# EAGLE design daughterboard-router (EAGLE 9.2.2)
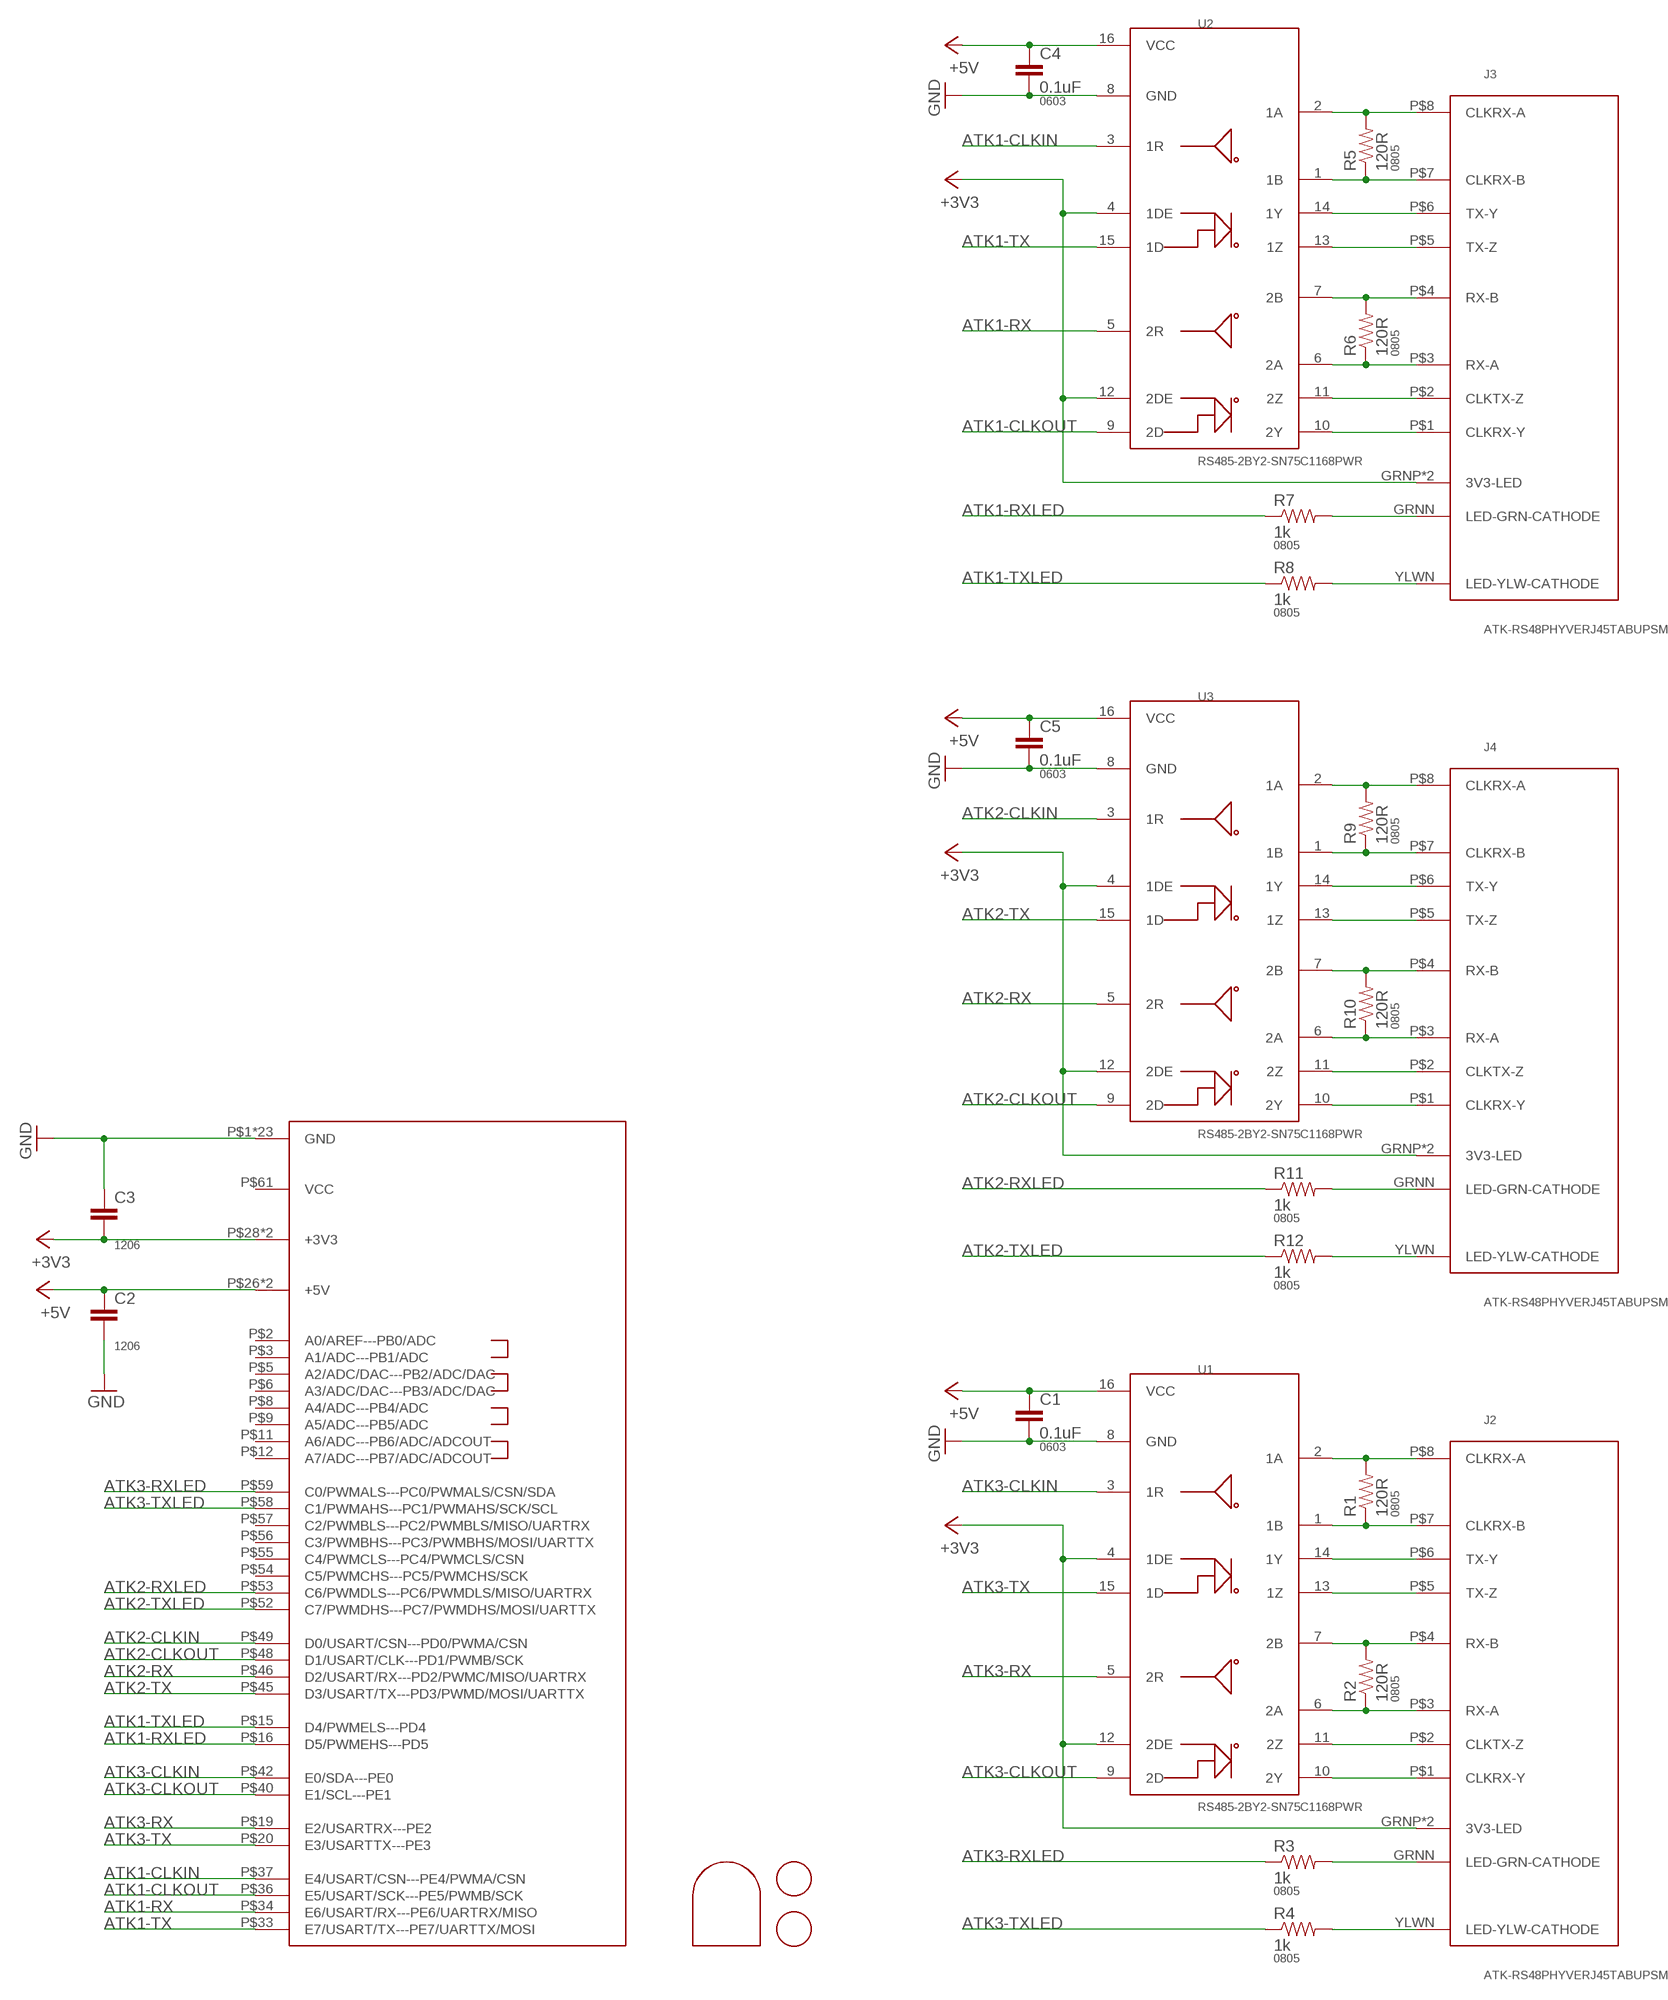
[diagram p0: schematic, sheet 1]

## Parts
C1  0.1uF  CAP0603-CAP  [0603-CAP]
C2  CAP1206  [1206]
C3  CAP1206  [1206]
C4  0.1uF  CAP0603-CAP  [0603-CAP]
C5  0.1uF  CAP0603-CAP  [0603-CAP]
J1  ATK-BFPPFX8-DAUGHTER  [ATK-BFPP-TOP-FX8-60]
J2  ATK-RS48PHYVERJ45TABUPSMD  [RJ45-LED-SMD-RJWURTH-634008137521]
J3  ATK-RS48PHYVERJ45TABUPSMD  [RJ45-LED-SMD-RJWURTH-634008137521]
J4  ATK-RS48PHYVERJ45TABUPSMD  [RJ45-LED-SMD-RJWURTH-634008137521]
J5  FIDUCIALRCT  [FIDUCIAL_RECT_1MM]
J6  FIDUCIALRCT  [FIDUCIAL_RECT_1MM]
MP1  JRTOMBSTONE  [JRTOMBSTONE]
R1  120R  RESISTOR0805-RES  [0805]
R2  120R  RESISTOR0805-RES  [0805]
R3  1k  RESISTOR0805-RES  [0805]
R4  1k  RESISTOR0805-RES  [0805]
R5  120R  RESISTOR0805-RES  [0805]
R6  120R  RESISTOR0805-RES  [0805]
R7  1k  RESISTOR0805-RES  [0805]
R8  1k  RESISTOR0805-RES  [0805]
R9  120R  RESISTOR0805-RES  [0805]
R10  120R  RESISTOR0805-RES  [0805]
R11  1k  RESISTOR0805-RES  [0805]
R12  1k  RESISTOR0805-RES  [0805]
U1  RS485-2BY2-SN75C1168PWR  [TSSOP16]
U2  RS485-2BY2-SN75C1168PWR  [TSSOP16]
U3  RS485-2BY2-SN75C1168PWR  [TSSOP16]

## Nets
+3V3: C3.2 J1.P$28(+3V3) J1.P$29(+3V3) J2.GRNP(3V3-LED) J2.YLWP(3V3-LED) J3.GRNP(3V3-LED) J3.YLWP(3V3-LED) J4.GRNP(3V3-LED) J4.YLWP(3V3-LED) U1.4(1DE) U1.12(2DE) U2.4(1DE) U2.12(2DE) U3.4(1DE) U3.12(2DE)
+5V: C1.1 C2.1 C4.1 C5.1 J1.P$26(+5V) J1.P$27(+5V) U1.16(VCC) U2.16(VCC) U3.16(VCC)
ATK1-CLKIN: J1.P$37(E4/USART/CSN---PE4/PWMA/CSN) U2.3(1R)
ATK1-CLKOUT: J1.P$36(E5/USART/SCK---PE5/PWMB/SCK) U2.9(2D)
ATK1-RX: J1.P$34(E6/USART/RX---PE6/UARTRX/MISO) U2.5(2R)
ATK1-RXLED: J1.P$16(D5/PWMEHS---PD5) R7.1
ATK1-TX: J1.P$33(E7/USART/TX---PE7/UARTTX/MOSI) U2.15(1D)
ATK1-TXLED: J1.P$15(D4/PWMELS---PD4) R8.1
ATK2-CLKIN: J1.P$49(D0/USART/CSN---PD0/PWMA/CSN) U3.3(1R)
ATK2-CLKOUT: J1.P$48(D1/USART/CLK---PD1/PWMB/SCK) U3.9(2D)
ATK2-RX: J1.P$46(D2/USART/RX---PD2/PWMC/MISO/UARTRX) U3.5(2R)
ATK2-RXLED: J1.P$53(C6/PWMDLS---PC6/PWMDLS/MISO/UARTRX) R11.1
ATK2-TX: J1.P$45(D3/USART/TX---PD3/PWMD/MOSI/UARTTX) U3.15(1D)
ATK2-TXLED: J1.P$52(C7/PWMDHS---PC7/PWMDHS/MOSI/UARTTX) R12.1
ATK3-CLKIN: J1.P$42(E0/SDA---PE0) U1.3(1R)
ATK3-CLKOUT: J1.P$40(E1/SCL---PE1) U1.9(2D)
ATK3-RX: J1.P$19(E2/USARTRX---PE2) U1.5(2R)
ATK3-RXLED: J1.P$59(C0/PWMALS---PC0/PWMALS/CSN/SDA) R3.1
ATK3-TX: J1.P$20(E3/USARTTX---PE3) U1.15(1D)
ATK3-TXLED: J1.P$58(C1/PWMAHS---PC1/PWMAHS/SCK/SCL) R4.1
GND: C1.2 C2.2 C3.1 C4.2 C5.2 J1.P$1(GND) J1.P$4(GND) J1.P$7(GND) J1.P$10(GND) J1.P$13(GND) J1.P$14(GND) J1.P$17(GND) J1.P$18(GND) J1.P$21(GND) J1.P$30(GND) J1.P$31(GND) J1.P$32(GND) J1.P$35(GND) J1.P$38(GND) J1.P$39(GND) J1.P$41(GND) J1.P$43(GND) J1.P$44(GND) J1.P$47(GND) J1.P$50(GND) J1.P$51(GND) J1.P$60(GND) J1.P$62(GND) U1.8(GND) U2.8(GND) U3.8(GND)
N$1: J3.P$4(RX-B) R6.2 U2.7(2B)
N$2: J2.P$4(RX-B) R2.2 U1.7(2B)
N$3: J2.P$3(RX-A) R2.1 U1.6(2A)
N$4: J2.P$5(TX-Z) U1.13(1Z)
N$5: J2.P$6(TX-Y) U1.14(1Y)
N$6: J2.P$7(CLKRX-B) R1.1 U1.1(1B)
N$7: J2.P$8(CLKRX-A) R1.2 U1.2(1A)
N$8: J2.P$2(CLKTX-Z) U1.11(2Z)
N$9: J2.P$1(CLKRX-Y) U1.10(2Y)
N$10: J3.P$3(RX-A) R6.1 U2.6(2A)
N$11: J2.GRNN(LED-GRN-CATHODE) R3.2
N$12: J2.YLWN(LED-YLW-CATHODE) R4.2
N$13: J3.P$5(TX-Z) U2.13(1Z)
N$14: J3.P$6(TX-Y) U2.14(1Y)
N$15: J3.P$7(CLKRX-B) R5.1 U2.1(1B)
N$16: J3.P$8(CLKRX-A) R5.2 U2.2(1A)
N$17: J3.P$2(CLKTX-Z) U2.11(2Z)
N$18: J3.P$1(CLKRX-Y) U2.10(2Y)
N$19: J3.GRNN(LED-GRN-CATHODE) R7.2
N$20: J3.YLWN(LED-YLW-CATHODE) R8.2
N$21: J4.P$4(RX-B) R10.2 U3.7(2B)
N$22: J4.P$3(RX-A) R10.1 U3.6(2A)
N$23: J4.P$5(TX-Z) U3.13(1Z)
N$24: J4.P$6(TX-Y) U3.14(1Y)
N$25: J4.P$7(CLKRX-B) R9.1 U3.1(1B)
N$26: J4.P$8(CLKRX-A) R9.2 U3.2(1A)
N$27: J4.P$2(CLKTX-Z) U3.11(2Z)
N$28: J4.P$1(CLKRX-Y) U3.10(2Y)
N$29: J4.GRNN(LED-GRN-CATHODE) R11.2
N$30: J4.YLWN(LED-YLW-CATHODE) R12.2
Unconnected: J1.P$2(A0/AREF---PB0/ADC) J1.P$3(A1/ADC---PB1/ADC) J1.P$5(A2/ADC/DAC---PB2/ADC/DAC) J1.P$6(A3/ADC/DAC---PB3/ADC/DAC) J1.P$8(A4/ADC---PB4/ADC) J1.P$9(A5/ADC---PB5/ADC) J1.P$11(A6/ADC---PB6/ADC/ADCOUT) J1.P$12(A7/ADC---PB7/ADC/ADCOUT) J1.P$54(C5/PWMCHS---PC5/PWMCHS/SCK) J1.P$55(C4/PWMCLS---PC4/PWMCLS/CSN) J1.P$56(C3/PWMBHS---PC3/PWMBHS/MOSI/UARTTX) J1.P$57(C2/PWMBLS---PC2/PWMBLS/MISO/UARTRX) J1.P$61(VCC)

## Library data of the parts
C1 C4 C5 = passives:CAP: Capacitor; PACKAGE: 0603
C2 C3 = passives:CAP: Capacitor; PACKAGE: 1206
J1 = connector:ATK-BFPP
J2-J4 = connector:ATK-RS48PHYVE
J5 J6 = connector:FIDUCIAL: For use by pick and place machines to calibrate the vision/machine, 1mm
MP1 = connector:JRTOMBSTONE
R1-R12 = passives:RESISTOR: Resistor; PACKAGE: 0805
U1-U3 = comm:RS485-2BY2-SN75C1168PWR

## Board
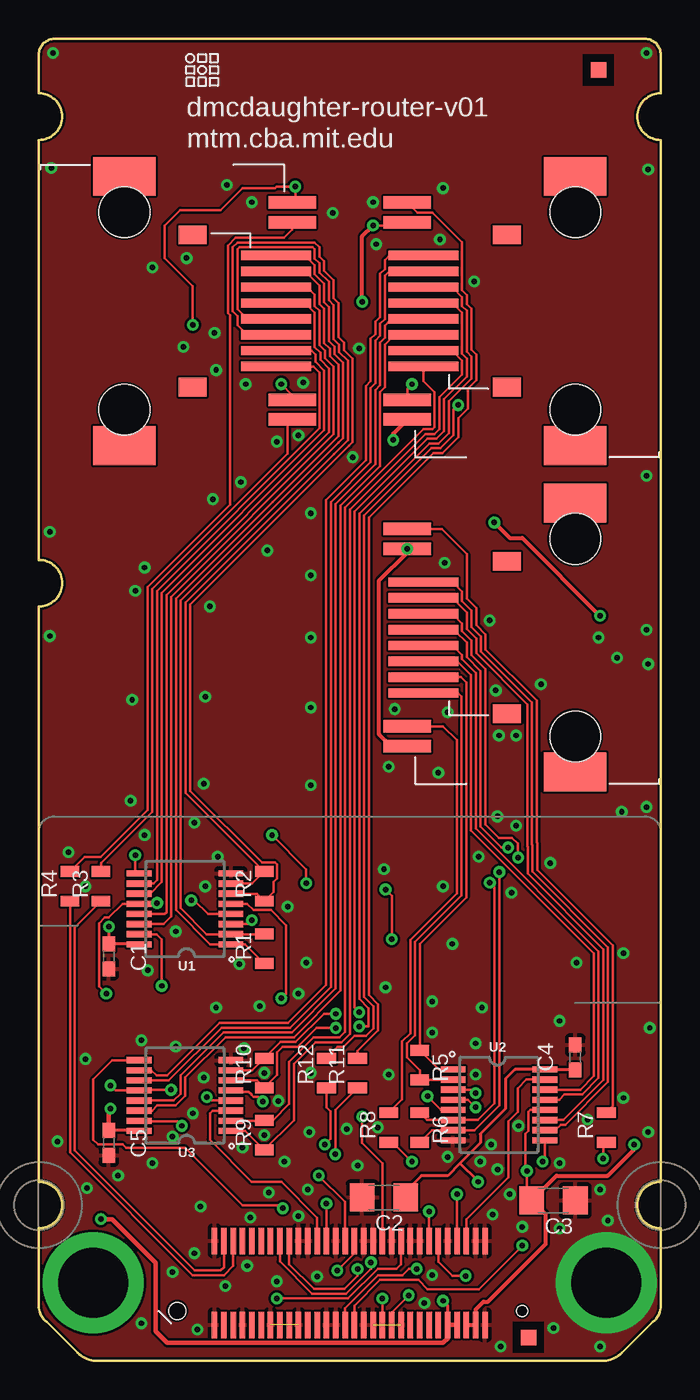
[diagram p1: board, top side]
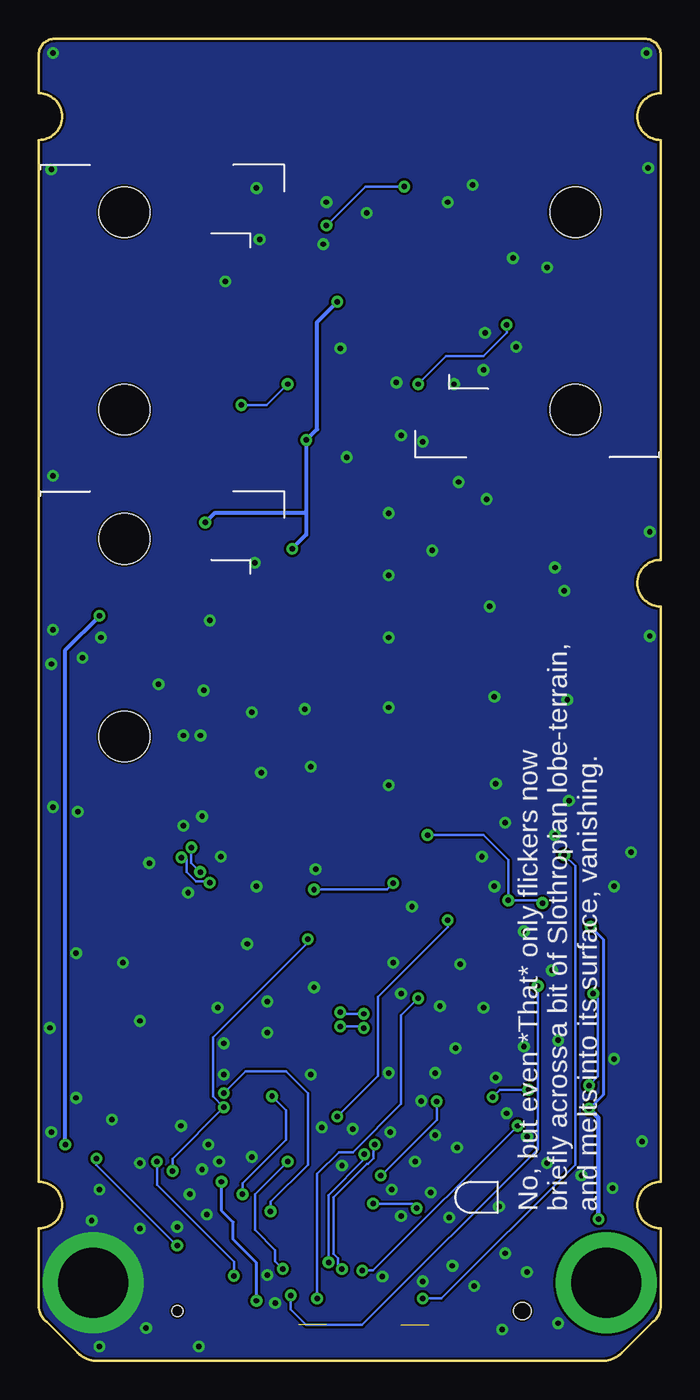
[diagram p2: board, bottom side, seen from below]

Size 40 x 85 mm. Coordinates in mm from the lower left corner, seen from the top.
Outline: 0,3.5 0,8.5 arc90 1.5,10 arc90 0,11.5 0,48.5 arc90 1.5,50 arc90 0,51.5 0,78.5 arc90 1.5,80 arc90 0,81.5 0,84 arc-90 1,85 39,85 arc-90 40,84 40,81.5 arc90 38.5,80 arc90 40,78.5 40,11.5 arc90 38.5,10 arc90 40,8.5 40,3.5 arc-53 39.5,2.5 37.5,0.5 arc-37 36.5,0 3.5,0 arc-37 2.5,0.5 0.5,2.5 arc-53 0,3.5
Copper layers (1*16): Top 0.035mm / dielectric 1.5mm / Bottom 0.035mm
Design rules "default *": minimum track width 6mil, minimum drill 0.35mm, track to track 6mil, track to pad 6mil, pad to pad 6mil, via to via 6mil, smd to smd 6mil, copper to edge 6mil, drill to drill 6mil, minimum pad ring 10mil, minimum via ring 8mil, stop-mask expansion 4mil, vias tented up to drill 30mil, thermal gap 10mil

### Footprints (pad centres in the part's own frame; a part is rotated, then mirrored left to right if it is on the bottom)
0603-CAP = smd 0.96 x 0.8: 1 -0.8,0; 2 0.8,0
1206 = smd 1.6 x 1.8: 1 -1.4,0; 2 1.4,0
ATK-BFPP-TOP-FX8-60 = smd 0.35 x 1.7: P$1 -8.7,-2.7; P$2 -8.1,-2.7; P$3 -7.5,-2.7; P$4 -6.9,-2.7; P$5 -6.3,-2.7; P$6 -5.7,-2.7; P$7 -5.1,-2.7; P$8 -4.5,-2.7; P$9 -3.9,-2.7; P$10 -3.3,-2.7; P$11 -2.7,-2.7; P$12 -2.1,-2.7; P$13 -1.5,-2.7; P$14 -0.9,-2.7; P$15 -0.3,-2.7; P$16 0.3,-2.7; P$17 0.9,-2.7; P$18 1.5,-2.7; P$19 2.1,-2.7; P$20 2.7,-2.7; P$21 3.3,-2.7; P$22 3.9,-2.7; P$23 4.5,-2.7; P$24 5.1,-2.7; P$25 5.7,-2.7; P$26 6.3,-2.7; P$27 6.9,-2.7; P$28 7.5,-2.7; P$29 8.1,-2.7; P$30 8.7,-2.7; P$31 8.7,2.7; P$32 8.1,2.7; P$33 7.5,2.7; P$34 6.9,2.7; P$35 6.3,2.7; P$36 5.7,2.7; P$37 5.1,2.7; P$38 4.5,2.7; P$39 3.9,2.7; P$40 3.3,2.7; P$41 2.7,2.7; P$42 2.1,2.7; P$43 1.5,2.7; P$44 0.9,2.7; P$45 0.3,2.7; P$46 -0.3,2.7; P$47 -0.9,2.7; P$48 -1.5,2.7; P$49 -2.1,2.7; P$50 -2.7,2.7; P$51 -3.3,2.7; P$52 -3.9,2.7; P$53 -4.5,2.7; P$54 -5.1,2.7; P$55 -5.7,2.7; P$56 -6.3,2.7; P$57 -6.9,2.7; P$58 -7.5,2.7; P$59 -8.1,2.7; P$60 -8.7,2.7 | drill 4.5 pad 6.5: P$61 -16.5,0; P$62 16.5,0 | hole 1.1: -11.1,-1.8 | hole 0.7: 11.1,-1.8
RJ45-LED-SMD-RJWURTH-634008137521 = smd 0.8 x 3.05: GRNN 6.98,10.8; GRNP 5.71,10.8; YLWN -5.71,10.8; YLWP -6.98,10.8 | smd 0.6 x 4.5: P$1 3.57,9.76; P$2 2.55,9.76; P$3 1.53,9.76; P$4 0.51,9.76; P$5 -0.51,9.76; P$6 -1.53,9.76; P$7 -2.55,9.76; P$8 -3.57,9.76 | smd 1.2 x 1.8: P$9 -4.9,4.4; P$10 4.9,4.4 | smd 2.5 x 4: P$13 -8.65,0; P$14 8.65,0 | hole 3.25: -6.35,0; 6.35,0
FIDUCIAL_RECT_1MM = smd 1 x 1: P$1 0,0
0805 = smd 0.7 x 1.2: 1 -0.95,0; 2 0.95,0
TSSOP16 = smd 0.4 x 1.6: 1 -2.225,-2.85; 2 -1.575,-2.85; 3 -0.925,-2.85; 4 -0.275,-2.85; 5 0.375,-2.85; 6 1.025,-2.85; 7 1.675,-2.85; 8 2.325,-2.85; 9 2.325,3.05; 10 1.675,3.05; 11 1.025,3.05; 12 0.375,3.05; 13 -0.275,3.05; 14 -0.925,3.05; 15 -1.575,3.05; 16 -2.225,3.05

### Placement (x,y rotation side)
C1  4.5,26 270 top
C2  22.2,10.5 180 top
C3  33.1,10.3 180 top
C4  34.5,19.5 90 top
C5  4.5,14 270 top
J1  20,5 0 top
J2  5.5,67.5 270 top
J3  34.5,46.5 90 top
J4  34.5,67.5 90 top
J5  36,83 0 top
J6  31.5,1.5 0 top
MP1  11.5,10.5 90 bottom
R1  14.5,26.5 90 top
R2  14.5,30.5 90 top
R3  4,30.5 90 top
R4  2,30.5 90 top
R5  24.5,19 270 top
R6  24.5,15 270 top
R7  36.5,15 90 top
R8  22.5,15 90 top
R9  14.5,14.5 90 top
R10  14.5,18.5 90 top
R11  20.5,18.5 90 top
R12  18.5,18.5 90 top
U1  9.5,29 90 top
U2  29.5,16.5 270 top
U3  9.5,17 90 top
U$1  CBA-LOGO  [CBA-SILK-LOGO]  10.5,83 0 top

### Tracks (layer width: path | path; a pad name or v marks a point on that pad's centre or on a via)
+3V3  (via drill 0.35)
  Top 0.152: J2.YLWP 16.5,74.68 v16.5,75.5 15.3,75.5 15.2,75.4 13.1,75.4 11.7,74 9.1,74 8.1,73 8.1,70.9 9.9,69.1 v9.9,66.6 | v21.5,73 23.49,73 J4.GRNP | v7.6,29.43 7.55,29.38 U1.12 5.38,29.38 4.51,28.51 4.25,28.51 3.87,28.13 3.87,24.06 v4.33,23.6 | v9.8,29.6 10,29.6 10.88,28.73 U1.4 | U2.4 27.62,16.77 v28.1,16.29 | C3.2 31.4,10.6 v31.4,12.2 31.3,12.3 31.3,14.57 31.5,14.77 31.5,16 31.62,16.12 U2.12 | U3.4 11.03,16.73 v10.8,16.95 | v4.6,17.7 4.92,17.38 U3.12 6.49,17.42 v8.51,17.42 | v22.7,27.1 22.7,29.9 v22.3,30.3 | v17.2,30.7 17.2,31.6 v15,33.8 | J2.GRNP 16.3,62.1 v15.6,62.8
  Top 0.254: J1.P$28 J1.P$29 28.1,3.3 28.6,3.8 28.9,3.8 32.6,7.5 32.6,9.4 C3.2 33.3,11.9 36.6,11.9 38.3,13.6 v38.3,13.9 | J3.YLWP 22.65,39.52 21.9,40.27 21.9,50.17 23.7,51.98 J3.GRNP | J4.YLWP 22.8,59.62 v22.8,59.2 | v20.8,68.1 20.8,72.3 v21.5,73 | v29.3,53.9 30.3,52.9 31.1,52.9 v36.1,47.9
  Bottom 0.152: v16.5,75.5 19,75.5 v21.5,73 | v7.6,29.43 7.78,29.6 v9.8,29.6 9.8,32.2 11.4,33.8 v15,33.8 | v31.4,12.2 31.4,12.99 v28.1,16.29 28.8,16.99 28.8,20.8 22.7,26.9 v22.7,27.1 | v4.6,17.7 4.03,18.27 4.03,23.3 v4.33,23.6 | v8.51,17.42 10.33,17.42 v10.8,16.95 | v22.3,30.3 17.6,30.3 v17.2,30.7 | v15.6,62.8 13.8,64.6 11.4,64.6 9.9,66.1 v9.9,66.6
  Bottom 0.254: v38.3,13.9 38.3,45.7 v36.1,47.9 | 22.8,54.5 v22.8,59.2 22.1,59.9 22.1,66.8 v20.8,68.1 | 22.8,54.5 22.8,53.11 J3.GRNP | 22.8,54.5 28.7,54.5 v29.3,53.9
  other vias: 23.7,52.21
+5V  (via drill 0.35)
  Top 0.152: 32.58,18.7 U2.16 | 23.6,10.9 C2.1
  Top 0.203: C4.1 32.58,18.7 | U2.16 30.62,18.73 30.03,18.13 30.03,16.2 28.4,14.57 28.4,14 27.1,12.7 | 27.1,12.7 26.3,11.9 24.6,11.9 23.6,10.9 | U3.16 6.42,14.8 C5.1 | v4.5,27.9 C1.1 6.42,26.8 U1.16 | J1.P$26 26.3,3.55 v26,3.85 | v28.25,11.5 28.25,11.55 27.1,12.7
  Top 0.305: J1.P$27 J1.P$26 26.3,1.44 26,1.15 8.26,1.15 7.5,1.9 7.5,6.3 4.7,9.1 v4,9.1 | v4.6,16.2 4.5,16.1 C5.1
  Bottom 0.203: v4.5,27.9 3.7,27.1 3.7,17.1 v4.6,16.2 | v26,3.85 26,6.3 27.5,7.8 27.5,8.9 28.25,9.65 v28.25,11.5
  Bottom 0.305: v4,9.1 4,15.6 v4.6,16.2
ATK1-CLKIN  (via drill 0.35)
  Top 0.152: U2.3 27.88,17.43 v28.1,17.2 | J1.P$37 v25.1,9.6
  Bottom 0.152: v25.1,9.6 25.1,10.2 22.7,12.6 22.7,17.2 24.1,18.6 26.7,18.6 v28.1,17.2
ATK1-CLKOUT  (via drill 0.35)
  Top 0.152: U2.9 32.55,12.95 v32.4,12.8 | J1.P$36 25.7,6.35 26.6,5.45 v27.45,5.45
  Bottom 0.152: v32.4,12.8 32.4,11.3 27.45,6.35 v27.45,5.45
ATK1-RX  (via drill 0.35)
  Top 0.152: U2.5 25.88,16.12 v25,17 | v26.9,10.7 J1.P$34
  Bottom 0.152: v25,17 24.1,16.1 24.1,14.2 26.9,11.4 v26.9,10.7
ATK1-RXLED  (via drill 0.35)
  Top 0.152: J1.P$16 20.3,3.54 21.96,5.2 24.41,5.2 25,4.6 28.3,4.6 v31.1,7.4 | v36.3,13 36.3,13.85 R7.1
  Bottom 0.152: v31.1,7.4 36.3,12.6 v36.3,13
ATK1-TX
  Top 0.152: J1.P$33 27.5,9.1 30.2,11.8 30.2,15.4 30.8,16 30.8,17.5 31.38,18.07 U2.15
ATK1-TXLED  (via drill 0.35)
  Top 0.152: R8.1 22.75,14.05 v24,12.8 | v24.3,5.9 23.8,5.9 23.4,5.5 21.83,5.5 19.7,3.37 J1.P$15
  Bottom 0.152: v24,12.8 26.1,10.7 26.1,8.4 24.8,7.1 24.8,6.4 v24.3,5.9
ATK2-CLKIN
  Top 0.152: U3.3 11.18,16.07 11,15.9 11,14.2 13.7,11.5 15.6,11.5 17.9,9.2 J1.P$49
ATK2-CLKOUT  (via drill 0.35)
  Top 0.152: J1.P$48 v18.5,10.1 | v15.7,9.8 15.5,10 13.1,10 9.4,13.7 5.6,13.7 5.39,13.91 4,13.91 4,13.9 3.8,13.9 3.5,14.2 3.5,18.1 4.72,19.32 U3.9
  Bottom 0.152: v18.5,10.1 16,10.1 v15.7,9.8
ATK2-RX  (via drill 0.35)
  Top 0.152: J1.P$46 19.7,10.2 v18,11.9 | v14.4,16.67 14.1,16.97 13.8,16.97 13.67,17.11 13.67,17.13 13.5,17.3 12.43,17.3 U3.5
  Bottom 0.152: v18,11.9 14.4,15.5 v14.4,16.67
ATK2-RXLED  (via drill 0.35)
  Top 0.152: R11.1 19.07,16.12 v19.07,13.27 | v21.36,6.32 21.36,5.89 19.77,4.3 17.57,4.3 15.5,6.38 J1.P$53
  Bottom 0.152: v19.07,13.27 19.07,12.93 21.36,10.64 v21.36,6.32
ATK2-TX  (via drill 0.35)
  Top 0.152: U3.15 6.47,15.4 8.9,15.4 v9.2,15.1 | v19.2,5.8 20.3,6.9 J1.P$45
  Bottom 0.152: v9.2,15.1 18.5,5.8 v19.2,5.8
ATK2-TXLED  (via drill 0.35)
  Top 0.152: R12.1 18.5,16.3 18.77,16.03 18.77,14.27 v18.4,13.9 | v20.5,5.89 20.5,5.46 19.65,4.61 17.7,4.61 16.1,6.21 J1.P$52
  Bottom 0.152: v18.4,13.9 18.46,13.84 18.46,13.02 18.82,12.66 18.91,12.66 21.06,10.51 21.06,6.87 20.75,6.57 20.75,6.14 v20.5,5.89
ATK3-CLKIN  (via drill 0.35)
  Top 0.152: U1.3 13.44,28.07 v13.7,28.33 | v20.8,15.7 20.8,14 22.1,12.7 J1.P$42
  Bottom 0.152: v13.7,28.33 13.7,27.9 18.2,23.4 18.2,18.3 v20.8,15.7
ATK3-CLKOUT  (via drill 0.35)
  Top 0.152: U1.9 6.2,31.57 v6.2,32.5 | v15.3,4 19.9,4 21.8,5.9 23,5.9 23.3,6.2 J1.P$40
  Bottom 0.152: v6.2,32.5 5.5,31.8 5.5,12.6 14.1,4 v15.3,4
ATK3-RX  (via drill 0.35)
  Top 0.152: J1.P$19 v22.1,4 | v15.6,23.3 15.9,23.6 15.9,28 14.93,28.97 13.8,28.97 13.4,29.38 U1.5
  Bottom 0.152: v15.6,23.3 16.7,22.2 16.7,16.5 19.8,13.4 20.7,13.4 22.1,12 v22.1,4
ATK3-RXLED
  Top 0.152: J1.P$59 11.9,6 11.71,5.8 10.03,5.8 2.31,13.53 2.31,27.86 R3.1
ATK3-TX  (via drill 0.35)
  Top 0.152: U1.15 7.58,27.43 7.9,27.1 v7.9,24.1 | J1.P$20 22.7,3.1 v23.8,4.2
  Bottom 0.152: v7.9,24.1 7.9,13.6 19.2,2.3 22.8,2.3 23.8,3.3 v23.8,4.2
ATK3-TXLED
  Top 0.152: R4.1 2,13.4 9.9,5.5 11.9,5.5 12.5,6.1 J1.P$58
GND  (via drill 0.35)  (2 unrouted)
  other vias: 20.6,65.1 20.2,58.1 26.6,26.8 11.5,32.4 17.5,54.5 17.5,50.5 17.5,46.5 17.5,42 17.5,37 13.2,20.1 15.4,16.7 14.5,18.5 14.5,14.5 17.5,18.5 16.7,23.6 17.2,25.6 19.8,14.9 14.8,10.8 10.4,9.9 7.3,12.7 8.8,20.2 6.6,20.6 30.85,15.1 33.5,21.85 20.5,12.55 10.6,18.2 9.9,15.9 10,6.9 5.1,11.9 3.1,11.1 3,19.4 1.2,14.1 3,30.5 8.8,27.6 10.7,30.5 10,34.6 16,29.2 12.9,25.5 7,25.1 14.2,22.8 22.3,24 22.2,31.6 26,30.5 28.3,32.4 25.3,21.1 28.5,22.7 22.5,18.4 17.4,14.7 13.1,13.7 15.8,12.8 17.3,11 16.7,9.3 13.6,9.2 13.4,6.1 12,4.8 6.6,2.4 10.2,2 17.9,5.4 15.3,5.1 24.8,3.7 25.3,5.5 21.8,15 25.3,23.1 28.1,20.4 28.1,18.4 30.4,30.1 32.9,32 37.6,26.2 37.6,16.9 35.3,15.5 33.5,12.7 36.1,11 39.2,14.7 33.5,8.5 31.1,8.6 33.1,2.1 29.7,0.9 36.1,0.9 36.6,9 29.5,12.3 29.1,13.9 28.4,12.8 26.3,13.1 29.2,9.4 30.3,10.7 8.6,5.7 8.6,14.4 11.4,22.7 5.9,36 1.9,32.7 6.8,33.8 10.6,37.1 6.8,51 6.2,49.5 11,48.5 14.7,52.1 10.7,42.7 6,42.5 11.2,55.4 13.3,62.8 17,62.9 15.3,59.1 13,56.5 28,69.4 25.8,72.1 21.7,71.8 21.5,74.5 26,75.4 18.9,73.8 13.7,74.5 12.1,75.6 9.5,70.9 7.3,70.3 9.3,65.2 11.3,66.1 11.4,63.7 29.4,43.1 29.6,40.2 30.7,34.4 30.7,40.2 29.5,35 26.3,41.7 22.9,41.9 26.1,51.3 16.7,59.5 0.7,46.6 0.7,53.3 0.8,76.7 0.9,84.1 39.1,84.1 39.2,76.6 39.1,56.9 39.1,47 37.2,45.2 39.2,44.8 36,46.5 37.5,35.3 39.1,35.6 39.3,21.4 34.6,25.6 32.3,43.5 29,47.6 25.7,37.8 22.5,38.2
  pour Top: -1,86 41,86 41,-1 -1,-1
  pour Bottom: -2,87 42,87 42,-2 -2,-2
N$1  (via drill 0.35)
  Top 0.152: J3.P$4 24.85,46.9 26.8,46.9 27.52,46.18 27.52,45.24 28.41,44.35 28.41,34.35 29.77,32.99 v30.2,32.99 | v29.62,31.42 29.62,16.42 28.02,14.82 U2.7 25.27,14.82 R6.2
  Bottom 0.152: v30.2,32.99 30.2,32 v29.62,31.42
N$2
  Top 0.152: U1.7 13.72,30.68 R2.2 9.43,36.52 9.43,48.74 18.99,58.3 | J2.P$4 13.4,67 12.78,67.61 12.78,71.47 12.91,71.6 17.61,71.6 17.74,71.47 17.74,70.88 18.04,70.57 18.04,69.98 18.65,69.37 18.65,68.19 18.96,67.89 18.96,65.7 19.32,65.33 19.32,64.86 19.88,64.3 19.88,59.2 18.99,58.3 | 18.99,58.3
N$3
  Top 0.152: U1.6 14.03,30.02 R2.1 15.1,30.15 15.1,30.78 15.33,31 15.33,31.89 15.2,32.03 14.35,32.03 9.73,36.65 9.73,48.62 19.96,58.84 | J2.P$3 13.41,65.97 12.78,66.59 12.78,67.18 12.48,67.49 12.48,71.59 12.79,71.9 17.73,71.9 18.04,71.59 18.04,71 18.35,70.7 18.35,70.11 18.96,69.5 18.96,68.32 19.26,68.02 19.26,65.82 19.63,65.46 19.63,64.99 20.19,64.43 20.19,59.07 19.96,58.84 | 19.96,58.84
N$4
  Top 0.152: U1.13 8.1,28.73 8.21,28.84 8.21,49.25 18.66,59.7 18.66,63.8 18.11,64.36 18.11,64.83 17.74,65.19 17.74,67.39 17.11,68.01 J2.P$5
N$5
  Top 0.152: J2.P$6 17.27,69.03 17.74,68.56 17.74,67.82 18.04,67.51 18.04,65.32 18.41,64.95 18.41,64.48 18.97,63.92 18.97,59.58 8.51,49.12 8.51,28.57 8.02,28.07 U1.14
N$6
  Top 0.152: R1.1 13.28,26.77 U1.1 11.03,26.77 8.82,28.98 8.82,48.99 15.02,55.2 | J2.P$7 17.11,70.05 18.04,69.12 18.04,67.94 18.35,67.64 18.35,65.44 18.71,65.08 18.71,64.61 19.27,64.05 19.27,59.45 15.02,55.2 | 15.02,55.2
N$7
  Top 0.152: R1.2 14.47,27.43 U1.2 10.81,27.43 9.12,29.11 9.12,48.87 19.28,59.02 | J2.P$8 17.11,71.07 17.74,70.44 17.74,69.86 18.35,69.25 18.35,68.07 18.65,67.76 18.65,65.57 19.02,65.2 19.02,64.74 19.58,64.18 19.58,59.32 19.28,59.02 | 19.28,59.02
N$8
  Top 0.152: U1.11 7.16,30.02 7.91,30.77 7.91,49.37 18.36,59.83 18.36,63.67 17.8,64.23 17.8,64.7 17.55,64.95 J2.P$2
N$9
  Top 0.152: J2.P$1 17.67,63.93 18.05,63.55 18.05,59.95 7.6,49.5 7.6,30.9 7.38,30.68 U1.10
N$10  (via drill 0.35)
  Top 0.152: R6.1 24.98,15.47 U2.6 28.24,15.47 29.32,16.55 29.32,30.44 v29.01,30.74 | v30.84,32.35 30.8,32.39 30.8,33.25 30.45,33.6 29.94,33.6 29.6,33.6 28.71,34.48 28.71,44.48 27.83,45.37 27.83,46.3 27.22,46.91 27.22,47.41 26.59,48.03 J3.P$3
  Bottom 0.152: v30.84,32.35 30.62,32.35 30.5,32.23 30.5,31.44 29.87,30.81 29.09,30.81 v29.01,30.74
N$11
  Top 0.152: J2.GRNN 16,60.22 16,58.33 7.29,49.63 7.29,35.3 4,32 R3.2
N$12
  Top 0.152: R4.2 2.95,32.4 3.97,32.4 6.99,35.42 6.99,49.75 12.3,55.06 12.3,67.23 12.17,67.36 12.17,71.72 12.66,72.21 15.78,72.21 16.3,72.73 J2.YLWN
N$13
  Top 0.152: J3.P$5 26.59,45.99 27.22,45.37 27.22,45.11 28.11,44.23 28.11,34.23 36.01,26.33 36.01,18.17 34.95,17.12 33.82,17.12 33.48,16.77 U2.13
N$14
  Top 0.152: J3.P$6 26.93,44.97 27.8,44.1 27.8,34.1 35.7,26.2 35.7,18.3 34.83,17.43 U2.14
N$15
  Top 0.152: 26.9,43.8 24.89,43.8 J3.P$7 27.15,43.95 27.5,43.6 27.5,29.8 24.5,26.8 R5.1 25.73,18.73 U2.1
N$16
  Top 0.152: 24.61,42.8 J3.P$8 26.97,42.93 27.19,42.71 27.19,29.92 24.2,26.93 24.2,20.92 23.67,20.39 23.67,19.5 24.5,18.68 R5.2 26.62,18.05 U2.2
N$17
  Top 0.152: J3.P$2 26.59,49.05 27.52,48.12 27.52,47.04 28.13,46.43 28.13,45.49 31.42,42.2 31.42,33.06 31.44,33.03 31.44,31.32 36.31,26.45 36.31,18.05 33.74,15.47 U2.11
N$18
  Top 0.152: U2.10 33.17,14.82 33.2,14.8 33.57,15.17 33.86,15.17 36.61,17.92 36.61,26.58 31.75,31.44 31.75,33.16 31.72,33.19 31.72,42.33 28.44,45.62 28.44,46.55 27.83,47.16 27.83,48.25 27.22,48.86 27.22,49.45 26.59,50.07 J3.P$1
N$19
  Top 0.152: J3.GRNN 25.92,53.48 27.52,51.88 27.52,49 28.13,48.39 28.13,47.29 28.74,46.68 28.74,45.74 32.03,42.46 32.03,33.31 32.05,33.29 32.05,31.57 36.92,26.7 36.92,16.37 R7.2
N$20
  Top 0.152: J3.YLWN 26.01,40.79 26.89,39.91 26.89,30.05 23.89,27.05 23.89,21.05 23.37,20.52 23.37,16.82 R8.2
N$21  (via drill 0.35)
  Top 0.152: U3.7 13.72,18.68 R10.2 15.54,20.5 16.53,20.5 18.33,22.3 v19.09,22.3 | J4.P$4 26.59,68.01 27.22,67.39 27.22,64.76 27.52,64.45 27.52,63.29 26.06,61.83 26.06,59.77 25.57,59.28 25,59.28 20.31,54.59 20.31,22.7 v20.61,22.4
  Bottom 0.152: v20.61,22.4 20.51,22.3 v19.09,22.3
N$22  (via drill 0.35)
  Top 0.152: U3.6 14.03,18.02 R10.1 15.33,18.38 15.33,19.83 15.69,20.19 16.65,20.19 17.85,21.39 v19.09,21.39 | v20.61,21.49 21.22,21.49 21.22,22.65 20.61,23.25 20.61,54.47 25.12,58.98 25.7,58.98 26.37,59.65 26.37,61.71 27.83,63.17 27.83,64.58 27.52,64.88 27.52,67.51 27.22,67.82 27.22,68.41 26.59,69.03 J4.P$3
  Bottom 0.152: v19.09,21.39 19.19,21.49 v20.61,21.49
N$23
  Top 0.152: J4.P$5 24.65,66.9 22.6,66.9 22.26,66.56 22.26,65.78 21.96,65.47 21.96,62.73 21.64,62.41 21.64,57.65 19.09,55.1 19.09,23.92 16.27,21.11 11.87,21.11 9.11,18.34 9.11,17.17 8.67,16.73 U3.13
N$24
  Top 0.152: J4.P$6 22.89,65.97 22.26,65.34 22.26,62.6 21.95,62.28 21.95,57.52 19.39,54.97 19.39,23.8 16.4,20.8 12,20.8 9.42,18.22 9.42,17.04 8.8,16.42 7.62,16.42 7.28,16.07 U3.14
N$25
  Top 0.152: U3.1 13.28,14.78 R9.1 16.41,15.46 16.41,19.08 17.8,20.48 19.47,20.48 20,21.01 20,54.72 24.87,59.59 25.45,59.59 25.76,59.9 25.76,61.96 27.22,63.42 27.22,64.33 26.59,64.95 J4.P$7
N$26
  Top 0.152: J4.P$8 24.74,63 25.45,62.28 25.45,60.02 25.32,59.89 24.75,59.89 19.7,54.85 19.7,21.14 19.34,20.78 17.68,20.78 16.1,19.21 16.1,16.5 15.05,15.45 R9.2 14.47,15.43 U3.2
N$27
  Top 0.152: J4.P$2 22.55,70.05 22.26,69.76 22.26,66.99 21.96,66.69 21.96,65.9 21.65,65.6 21.65,62.85 21.34,62.54 21.34,57.78 18.79,55.23 18.79,24.05 16.15,21.41 11.75,21.41 8.36,18.02 U3.11
N$28
  Top 0.152: U3.10 7.22,18.68 7.57,18.33 8.24,18.33 11.62,21.71 16.02,21.71 18.48,24.17 18.48,55.35 21.03,57.9 21.03,62.66 21.35,62.98 21.35,65.72 21.65,66.03 21.65,66.81 21.96,67.12 21.96,69.89 22.26,70.19 22.26,70.76 22.5,71 24.67,71 J4.P$1
N$29
  Top 0.152: J4.GRNN 24.34,73.84 25.32,73.84 27.22,71.94 27.22,68.84 27.52,68.53 27.52,67.94 27.83,67.64 27.83,65.01 28.13,64.7 28.13,63.04 27.6,62.51 27.6,61.22 26.98,60.6 26.98,59.39 25.95,58.37 25.38,58.37 21.22,54.22 21.22,23.51 21.83,22.9 21.83,21.24 20.5,19.91 R11.2
N$30  (via drill 0.35)
  Top 0.152: R12.2 19.23,20.18 19.6,20.18 20.31,20.88 21.04,20.88 21.52,21.36 21.52,22.78 20.92,23.38 20.92,54.34 25.25,58.67 25.82,58.67 26.67,59.52 26.67,61.15 v26.98,61.45 | J4.YLWN 23.7,62.5 v24,62.8
  Bottom 0.152: v24,62.8 25.34,61.45 v26.98,61.45

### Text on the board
tPlace: dmcdaughter-router-v01 | mtm.cba.mit.edu
bPlace: No, but even *That* only flickers now / briefly across a bit of Slothropian lobe-terrain, / and melts into its surface, vanishing.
